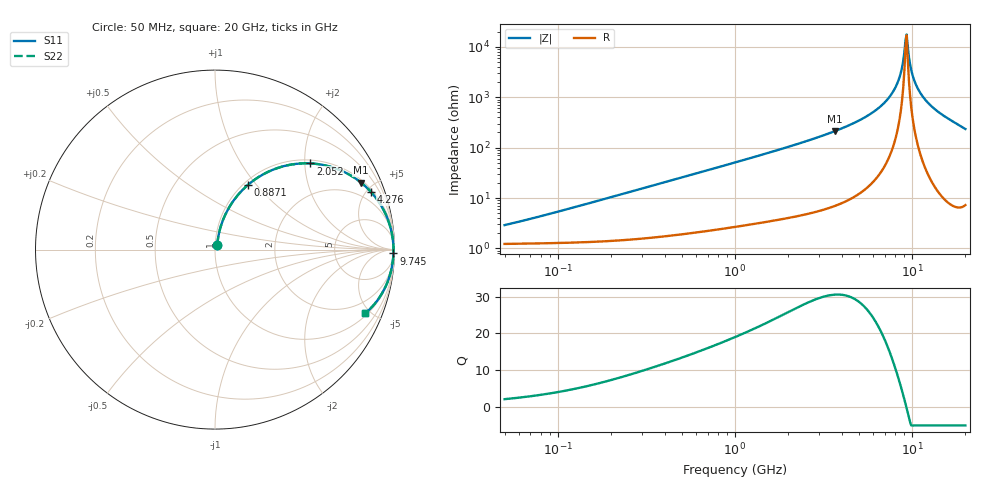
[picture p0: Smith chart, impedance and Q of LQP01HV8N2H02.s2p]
!Murata Part Number: LQP01HV8N2H02
!These Parameters are Measured in Series Mode Connection
!  o--[Z]--o
!Port1  Port2
!  o-------o
!Freq. Start=50[MHz] Stop=20[GHz], 401[Steps]
# Hz S RI R 50
!Freq.(Hz) S11(Real) S11(Imag) S21(Real) S21(Imag) S12(Real) S12(Imag) S22(Real) S22(Imag)
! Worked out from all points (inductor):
!   401 points, 50 MHz to 20 GHz, reference 50 ohm
!   read as one part in series: L = 8.3 nH near 72.71 MHz
!   highest Q = 30.5 at 3.681 GHz (marker M1), where L = 9.26 nH
!   self-resonance near 9.178 GHz
!   S11 on the Smith chart (normalised r, x): 50 MHz: 1.02, +0.05; 887.1 MHz: 1.05, +0.90; 2.052 GHz: 1.08, +2.13; 4.276 GHz: 1.18, +5.31; 9.745 GHz: 22, -87; 20 GHz: 1.14, -4.68
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5e7  0.0128 0.0256  0.9872 -0.0256  0.9872 -0.0256  0.0128 0.0256
1.364002e8  0.0179 0.0687  0.9821 -0.0687  0.9821 -0.0687  0.0179 0.0687
3.721004e8  0.0501 0.1782  0.9499 -0.1782  0.9499 -0.1782  0.0501 0.1782
8.870719e8  0.182 0.359  0.818 -0.359  0.818 -0.359  0.182 0.359
1e9  0.217 0.3867  0.783 -0.3867  0.783 -0.3867  0.217 0.3867
2.05233e9  0.5313 0.4802  0.4687 -0.4802  0.4687 -0.4802  0.5313 0.4802
2.728004e9  0.6779 0.4503  0.3221 -0.4503  0.3221 -0.4503  0.6779 0.4503
3.680849e9  0.8132 0.3737  0.1868 -0.3737  0.1868 -0.3737  0.8132 0.3737
4.275624e9  0.8678 0.3225  0.1322 -0.3225  0.1322 -0.3225  0.8678 0.3225
5.944466e9  0.953 0.1924  0.047 -0.1924  0.047 -0.1924  0.953 0.1924
7.442007e9  0.984 0.0967  0.016 -0.0967  0.016 -0.0967  0.984 0.0967
8.389408e9  0.9922 0.0445  0.00783 -0.0445  0.00783 -0.0445  0.9922 0.0445
8.644534e9  0.9933 0.0314  0.00669 -0.0314  0.00669 -0.0314  0.9933 0.0314
9.041845e9  0.9943 0.0116  0.00565 -0.0116  0.00565 -0.0116  0.9943 0.0116
9.178299e9  0.9945 0.00502  0.00549 -0.00502  0.00549 -0.00502  0.9945 0.00502
9.457416e9  0.9946 -0.0082  0.00542 0.0082  0.00542 0.0082  0.9946 -0.0082
9.745021e9  0.9943 -0.0215  0.00572 0.0215  0.00572 0.0215  0.9943 -0.0215
1.004137e10  0.9936 -0.0347  0.00638 0.0347  0.00638 0.0347  0.9936 -0.0347
1.050288e10  0.9919 -0.0547  0.00807 0.0547  0.00807 0.0547  0.9919 -0.0547
1.201863e10  0.9817 -0.115  0.0183 0.115  0.0183 0.115  0.9817 -0.115
1.460232e10  0.9514 -0.2034  0.0486 0.2034  0.0486 0.2034  0.9514 -0.2034
2e10  0.8382 -0.3531  0.1618 0.3531  0.1618 0.3531  0.8382 -0.3531
